|Texas Instruments Incorporated
|IWR6843AOP Single-Chip 60- to 64-GHz mmWave Sensor
[IBIS Ver]   4.1
[File name]   xwr6843aop_fcbga180.ibs
[Date]   04/01/2020
[File Rev]   1.0
[Source]
| Texas Instruments Incorporated.
| Analog-eLab Design Center, HPA
| 12500 TI Blvd
| Dallas, TX -75243
[Notes]   Revision History:
| Rev 1.0: 04/01/2020
| - Initial version of the model
| - C_comp although listed in numerical order of value are
|   obtained from varying PVT conditions. For PVT conditions for
|   each specific value refer the buffer description under
|   respective [Model]. IBIS model user is responsible for using
|   appropriate C_comp to simulate for Signal Integrity.
[Disclaimer]
| This model is designed as an aid for customers of Texas Instruments.
| TI and its licensors and suppliers make no warranties, either expressed
| or implied, with respect to this  model, including the warranties of
| merchantability or fitness for a particular purpose. The model is
| provided solely on an "as is" basis. The entire risk as to its quality
| and performance is with the customer.
| This model is subject to change without notice. Texas Instruments
| Incorporated is not responsible for updating this model.
[Copyright]
(C) Copyright 2018 Texas Instruments Incorporated.All rights reserved.
|  Component XI6843ARQGALP 180-pin FCBGA -ALP0180 package
|  Part # XI6843ARQGALP
[Component]   XI6843ARQGALP
[Manufacturer]   Texas Instruments
[Package]   |180 FCBGA - ALP0180 package
|  variable   typ   min   max
R_pkg   0.26   0.10   0.58
L_pkg   2.4nH   1.1nH   4.4nH
C_pkg   0.5pF   0.18pF   1.7pF
[Pin]   signal_name   model_name   R_pin   L_pin   C_pin
A1   VSS   GND   NA   NA   NA
A2   VSS   GND   NA   NA   NA
A3   DP11   IO1   NA   NA   NA
A4   DP13   IO1   NA   NA   NA
A5   VIN_SRAM   POWER   NA   NA   NA
A6   VSSA   GND   NA   NA   NA
A7   CLKP   NC   NA   NA   NA
A8   VSSA   GND   NA   NA   NA
A9   VOUT_14SYNTH   NC   NA   NA   NA
A10   VOUT_14APLL   NC   NA   NA   NA
A11   VSSA   GND   NA   NA   NA
A12   VIN_18VCO   POWER   NA   NA   NA
A13   VSSA   GND   NA   NA   NA
A14   OSC_CLKOUT   NC   NA   NA   NA
A15   VSSA   GND   NA   NA   NA
A16   VBGAP   NC   NA   NA   NA
A17   VSSA   GND   NA   NA   NA
A18   VSSA   GND   NA   NA   NA
B1   VIOIN_18   POWER   NA   NA   NA
B2   SPI_HOST_INTR   NC   NA   NA   NA
B3   DP9   IO1   NA   NA   NA
B4   DP12   IO1   NA   NA   NA
B5   DP15   IO1   NA   NA   NA
B6   VSSA   GND   NA   NA   NA
B7   CLKM   NC   NA   NA   NA
B8   VSSA   GND   NA   NA   NA
B9   VSSA   GND   NA   NA   NA
B10   VSSA   GND   NA   NA   NA
B11   VSSA   GND   NA   NA   NA
B12   VSSA   GND   NA   NA   NA
B13   VSSA   GND   NA   NA   NA
B14   VSSA   GND   NA   NA   NA
B15   VSSA   GND   NA   NA   NA
B16   VSSA   GND   NA   NA   NA
B17   VSSA   GND   NA   NA   NA
B18   VSSA   GND   NA   NA   NA
C1   VNWA   POWER   NA   NA   NA
C2   SPIA_CS_N   IO1   NA   NA   NA
C3   DP8   IO1   NA   NA   NA
C4   DP10   IO1   NA   NA   NA
C5   DP14   IO1   NA   NA   NA
C6   VSSA   GND   NA   NA   NA
C7   VSSA   GND   NA   NA   NA
C8   VSSA   GND   NA   NA   NA
C9   GPADC_5   NC   NA   NA   NA
C10   GPADC_6   NC   NA   NA   NA
C11   VIN_18VCO   POWER   NA   NA   NA
C12   VSSA   GND   NA   NA   NA
C13   VSSA   GND   NA   NA   NA
C14   VSSA   GND   NA   NA   NA
C15   VIN_18CLK   POWER   NA   NA   NA
C16   VSSA   GND   NA   NA   NA
C17   VSSA   GND   NA   NA   NA
C18   VIN_18CLK   POWER   NA   NA   NA
D1   SPIA_MISO   IO2   NA   NA   NA
D2   SPIA_CLK   IO2   NA   NA   NA
D3   SPIB_CS_N   IO2   NA   NA   NA
D16   VSSA   GND   NA   NA   NA
D17   VSSA   GND   NA   NA   NA
D18   VSSA   GND   NA   NA   NA
E1   VDDIN   POWER   NA   NA   NA
E2   SPIB_CLK   IO2   NA   NA   NA
E3   VSS   GND   NA   NA   NA
E16   VSSA   GND   NA   NA   NA
E17   VSSA   GND   NA   NA   NA
E18   VSSA   GND   NA   NA   NA
F1   VIOIN_18   POWER   NA   NA   NA
F2   SPIA_MOSI   IO2   NA   NA   NA
F3   VSS   GND   NA   NA   NA
F16   VSSA   GND   NA   NA   NA
F17   VSSA   GND   NA   NA   NA
F18   VSSA   GND   NA   NA   NA
G1   SPIB_MOSI   IO2   NA   NA   NA
G2   QSPI[1]   IO2   NA   NA   NA
G3   SPIB_MISO   IO2   NA   NA   NA
G16   VOUT_PA   NC   NA   NA   NA
G17   VOUT_PA   NC   NA   NA   NA
G18   VOUT_PA   NC   NA   NA   NA
H1   VIOIN   POWER   NA   NA   NA
H2   QSPI_CLK   IO2   NA   NA   NA
H3   QSPI[0]   IO2   NA   NA   NA
H16   VIN_13RF2   POWER   NA   NA   NA
H17   VIN_13RF2   POWER   NA   NA   NA
H18   VIN_13RF2   POWER   NA   NA   NA
J1   VDDIN   POWER   NA   NA   NA
J2   QSPI_CS_N   IO1   NA   NA   NA
J3   QSPI[2]   IO2   NA   NA   NA
J16   VIN_13RF1   POWER   NA   NA   NA
J17   VIN_13RF1   POWER   NA   NA   NA
J18   VIN_13RF1   POWER   NA   NA   NA
K1   VIOIN_18   POWER   NA   NA   NA
K2   QSPI[3]   IO2   NA   NA   NA
K3   GPIO_2   IO2   NA   NA   NA
K16   VSSA   GND   NA   NA   NA
K17   VSSA   GND   NA   NA   NA
K18   VSSA   GND   NA   NA   NA
L1   DP7   IO2   NA   NA   NA
L2   DP6   IO2   NA   NA   NA
L3   GPIO_1   IO2   NA   NA   NA
L16   VSSA   GND   NA   NA   NA
L17   VSSA   GND   NA   NA   NA
L18   VSSA   GND   NA   NA   NA
M1   DP5   IO2   NA   NA   NA
M2   GPIO_0   IO2   NA   NA   NA
M3   SYNC_OUT   IO2   NA   NA   NA
M16   VIN_18BB   POWER   NA   NA   NA
M17   VIN_18BB   POWER   NA   NA   NA
M18   VIN_18BB   POWER   NA   NA   NA
N1   LVDS_TXM[0]   ODF   NA   NA   NA
N2   LVDS_TXP[0]   ODF   NA   NA   NA
N3   VSS   GND   NA   NA   NA
N16   VSSA   GND   NA   NA   NA
N17   VSSA   GND   NA   NA   NA
N18   VSSA   GND   NA   NA   NA
P1   LVDS_TXM[1]   ODF   NA   NA   NA
P2   LVDS_TXP[1]   ODF   NA   NA   NA
P3   VSS   GND   NA   NA   NA
P16   VSSA   GND   NA   NA   NA
P17   GPADC_2   NC   NA   NA   NA
P18   GPADC_1   NC   NA   NA   NA
R1   LVDS_CLKP   ODF   NA   NA   NA
R2   LVDS_CLKM   ODF   NA   NA   NA
R3   VSS   GND   NA   NA   NA
R16   VSSA   GND   NA   NA   NA
R17   VSSA   GND   NA   NA   NA
R18   GPADC_3   NC   NA   NA   NA
T1   LVDS_FRCLKP   ODF   NA   NA   NA
T2   LVDS_FRCLKM   ODF   NA   NA   NA
T3   TCK   IO2   NA   NA   NA
T4   VSS   GND   NA   NA   NA
T5   VSS   GND   NA   NA   NA
T6   VSS   GND   NA   NA   NA
T7   VSS   GND   NA   NA   NA
T8   VSS   GND   NA   NA   NA
T9   VSS   GND   NA   NA   NA
T10   VSS   GND   NA   NA   NA
T11   VSS   GND   NA   NA   NA
T12   VSS   GND   NA   NA   NA
T13   VSS   GND   NA   NA   NA
T14   VSS   GND   NA   NA   NA
T15   VSS   GND   NA   NA   NA
T16   VSS   GND   NA   NA   NA
T17   VSSA   GND   NA   NA   NA
T18   GPADC_4   NC   NA   NA   NA
U1   VSS   GND   NA   NA   NA
U2   VIOIN_18DIFF   POWER   NA   NA   NA
U3   DMM_CLK   IO1   NA   NA   NA
U4   DMM_SYNC   IO1   NA   NA   NA
U5   DP3   IO1   NA   NA   NA
U6   DP1   IO1   NA   NA   NA
U7   DP0   IO1   NA   NA   NA
U8   TMS   IO1   NA   NA   NA
U9   TDI   IO1   NA   NA   NA
U10   TDO   IO1   NA   NA   NA
U11   NRESET   NC   NA   NA   NA
U12   SYNC_IN   IO1   NA   NA   NA
U13   WARM_RESET   IOOD   NA   NA   NA
U14   NERROR_IN   IOOD   NA   NA   NA
U15   NERROR_OUT   IOOD   NA   NA   NA
U16   RS232_TX   IO1   NA   NA   NA
U17   VSSA   GND   NA   NA   NA
U18   VSSA   GND   NA   NA   NA
V1   VSS   GND   NA   NA   NA
V2   VPP   POWER   NA   NA   NA
V3   DP4   IO1   NA   NA   NA
V4   VDDIN   POWER   NA   NA   NA
V5   DP2   IO1   NA   NA   NA
V6   VIN_SRAM   POWER   NA   NA   NA
V7   VNWA   POWER   NA   NA   NA
V8   VDDIN   POWER   NA   NA   NA
V9   VIOIN   POWER   NA   NA   NA
V10   PMIC_CLKOUT   IO1   NA   NA   NA
V11   VIOIN_18   POWER   NA   NA   NA
V12   VIN_SRAM   POWER   NA   NA   NA
V13   MCU_CLKOUT   IO1   NA   NA   NA
V14   VNWA   POWER   NA   NA   NA
V15   VDDIN   POWER   NA   NA   NA
V16   RS232_RX   IO1   NA   NA   NA
V17   VSSA   GND   NA   NA   NA
V18   VSSA   GND   NA   NA   NA
[Diff Pin]  inv_pin  vdiff  tdelay_typ  tdelay_min  tdelay_max
   N1   N2   0.1   NA   NA   NA
   P1   P2   0.1   NA   NA   NA
   R2   R1   0.1   NA   NA   NA
   T2   T1   0.1   NA   NA   NA
| Model IOOD
[Model Selector] IOOD
|SC1 IS A SLEW RATE CONTROL PIN
|5% SUPPLY VARIATION MODES WITH 1.8V NOM SUPPLY
IOOD_V_PUPDOFF_5P_SC1_1P8  Cell operated at 1.8(nom)
|IOOD_V_PUPDOFF_5P_SC1_1P8; BUFFER WITH WEAK PULUP/PULLDOWN OFF AT 5% SUPPLY
|VARIATION WITH SC1=1 MEANING SLOW MODE OF OPERATION
IOOD_V_PD_ON_5P_!SC1_1P8  Cell operated at 1.8(nom)
|IOOD_V_PD_ON_5P_!SC1_1P8; BUFFER WITH WEAK_PULLDOWN_ON AT 5% SUPPLY
|VARIATION WITH SC1=0 MEANING FAST MODE OF OPERATION
IOOD_V_PD_ON_5P_SC1_1P8  Cell operated at 1.8(nom)
|IOOD_V_PD_ON_5P_SC1_1P8; BUFFER WITH WEAK_PULLDOWN_ON AT 5% SUPPLY
|VARIATION WITH SC1=1 MEANING SLOW MODE OF OPERATION
IOOD_V_PU_ON_5P_!SC1_1P8  Cell operated at 1.8(nom)
|IOOD_V_PU_ON_5P_!SC1_1P8; BUFFER WITH WEAK_PULLUP_ON AT 5% SUPPLY
|VARIATION WITH SC1=0 MEANING FAST MODE OF OPERATION
IOOD_V_PUPDOFF_5P_!SC1_1P8  Cell operated at 1.8(nom)
|IOOD_V_PUPDOFF_5P_!SC1_1P8; BUFFER WITH WEAK PULUP/PULLDOWN OFF AT 5% SUPPLY
|VARIATION WITH SC1=0 MEANING FAST MODE OF OPERATION
IOOD_V_PU_ON_5P_SC1_1P8  Cell operated at 1.8(nom)
|IOOD_V_PU_ON_5P_SC1_1P8; BUFFER WITH WEAK_PULLUP_ON AT 5% SUPPLY
|VARIATION WITH SC1=1 MEANING SLOW MODE OF OPERATION
|5% SUPPLY VARIATION MODES WITH 3.3V NOM SUPPLY
IOOD_V_PUPDOFF_5P_SC1_3P3  Cell operated at 3.3(nom)
|IOOD_V_PUPDOFF_5P_SC1_3P3; BUFFER WITH WEAK PULUP/PULLDOWN OFF AT 5% SUPPLY
|VARIATION WITH SC1=1 MEANING SLOW MODE OF OPERATION
IOOD_V_PD_ON_5P_!SC1_3P3  Cell operated at 3.3(nom)
|IOOD_V_PD_ON_5P_!SC1_3P3; BUFFER WITH WEAK_PULLDOWN_ON AT 5% SUPPLY
|VARIATION WITH SC1=0 MEANING FAST MODE OF OPERATION
IOOD_V_PD_ON_5P_SC1_3P3  Cell operated at 3.3(nom)
|IOOD_V_PD_ON_5P_SC1_3P3; BUFFER WITH WEAK_PULLDOWN_ON AT 5% SUPPLY
|VARIATION WITH SC1=1 MEANING SLOW MODE OF OPERATION
IOOD_V_PU_ON_5P_!SC1_3P3  Cell operated at 3.3(nom)
|IOOD_V_PU_ON_5P_!SC1_3P3; BUFFER WITH WEAK_PULLUP_ON AT 5% SUPPLY
|VARIATION WITH SC1=0 MEANING FAST MODE OF OPERATION
IOOD_V_PUPDOFF_5P_!SC1_3P3  Cell operated at 3.3(nom)
|IOOD_V_PUPDOFF_5P_!SC1_3P3; BUFFER WITH WEAK PULUP/PULLDOWN OFF AT 5% SUPPLY
|VARIATION WITH SC1=0 MEANING FAST MODE OF OPERATION
IOOD_V_PU_ON_5P_SC1_3P3  Cell operated at 3.3(nom)
|IOOD_V_PU_ON_5P_SC1_3P3; BUFFER WITH WEAK_PULLUP_ON AT 5% SUPPLY
|VARIATION WITH SC1=1 MEANING SLOW MODE OF OPERATION
| 10% SUPPLY VARIATION MODES WITH 1.8V NOM SUPPLY
IOOD_V_PUPDOFF_10P_SC1_1P8  Cell operated at 1.8(nom)
|IOOD_V_PUPDOFF_10P_SC1_1P8; BUFFER WITH WEAK PULUP/PULLDOWN OFF AT 10% SUPPLY
|VARIATION WITH SC1=1 MEANING SLOW MODE OF OPERATION
IOOD_V_PD_ON_10P_!SC1_1P8  Cell operated at 1.8(nom)
|IOOD_V_PD_ON_10P_!SC1_1P8; BUFFER WITH WEAK_PULLDOWN_ON AT 10% SUPPLY
|VARIATION WITH SC1=0 MEANING FAST MODE OF OPERATION
IOOD_V_PD_ON_10P_SC1_1P8  Cell operated at 1.8(nom)
|IOOD_V_PD_ON_10P_SC1_1P8; BUFFER WITH WEAK_PULLDOWN_ON AT 10% SUPPLY
|VARIATION WITH SC1=1 MEANING SLOW MODE OF OPERATION
IOOD_V_PU_ON_10P_!SC1_1P8  Cell operated at 1.8(nom)
|IOOD_V_PU_ON_10P_!SC1_1P8; BUFFER WITH WEAK_PULLUP_ON AT 10% SUPPLY
|VARIATION WITH SC1=0 MEANING FAST MODE OF OPERATION
IOOD_V_PUPDOFF_10P_!SC1_1P8  Cell operated at 1.8(nom)
|IOOD_V_PUPDOFF_10P_!SC1_1P8; BUFFER WITH WEAK PULUP/PULLDOWN OFF AT 10% SUPPLY
|VARIATION WITH SC1=0 MEANING FAST MODE OF OPERATION
IOOD_V_PU_ON_10P_SC1_1P8  Cell operated at 1.8(nom)
|IOOD_V_PU_ON_10P_SC1_1P8; BUFFER WITH WEAK_PULLUP_ON AT 10% SUPPLY
|VARIATION WITH SC1=1 MEANING SLOW MODE OF OPERATION
| 10% SUPPLY VARIATION MODES WITH 3.3V NOM SUPPLY
IOOD_V_PUPDOFF_10P_SC1_3P3  Cell operated at 3.3(nom)
|IOOD_V_PUPDOFF_10P_SC1_3P3; BUFFER WITH WEAK PULUP/PULLDOWN OFF AT 10% SUPPLY
|VARIATION WITH SC1=1 MEANING SLOW MODE OF OPERATION
IOOD_V_PD_ON_10P_!SC1_3P3  Cell operated at 3.3(nom)
|IOOD_V_PD_ON_10P_!SC1_3P3; BUFFER WITH WEAK_PULLDOWN_ON 10% SUPPLY
|VARIATION WITH SC1=0 MEANING FAST MODE OF OPERATION
IOOD_V_PD_ON_10P_SC1_3P3  Cell operated at 3.3(nom)
|IOOD_V_PD_ON_10P_SC1_3P3; BUFFER WITH WEAK_PULLDOWN_ON AT 10% SUPPLY
|VARIATION WITH SC1=1 MEANING SLOW MODE OF OPERATION
IOOD_V_PU_ON_10P_!SC1_3P3  Cell operated at 3.3(nom)
|IOOD_V_PU_ON_10P_!SC1_3P3; BUFFER WITH WEAK_PULLUP_ON AT 10% SUPPLY
|VARIATION WITH SC1=0 MEANING FAST MODE OF OPERATION
IOOD_V_PUPDOFF_10P_!SC1_3P3  Cell operated at 3.3(nom)
|IOOD_V_PUPDOFF_10P_!SC1_3P3; BUFFER WITH WEAK PULUP/PULLDOWN OFF AT 10% SUPPLY
|VARIATION WITH SC1=0 MEANING FAST MODE OF OPERATION
IOOD_V_PU_ON_10P_SC1_3P3  Cell operated at 3.3(nom)
|IOOD_V_PU_ON_10P_SC1_3P3; BUFFER WITH WEAK_PULLUP_ON AT 10% SUPPLY
|VARIATION WITH SC1=1 MEANING SLOW MODE OF OPERATION
| Model IO1
[Model Selector] IO1
|SC1 IS A SLEW RATE CONTROL PIN
|5% SUPPLY VARIATION MODES WITH 1.8V NOM SUPPLY
IO1_V_PUPDOFF_5P_SC1_1P8  Cell operated at 1.8(nom)
|IO1_V_PUPDOFF_5P_SC1_1P8; BUFFER WITH WEAK PULUP/PULLDOWN OFF AT 5% SUPPLY
|VARIATION WITH SC1=1 MEANING SLOW MODE OF OPERATION
IO1_V_PD_ON_5P_!SC1_1P8  Cell operated at 1.8(nom)
|IO1_V_PD_ON_5P_!SC1_1P8; BUFFER WITH WEAK_PULLDOWN_ON AT 5% SUPPLY
|VARIATION WITH SC1=0 MEANING FAST MODE OF OPERATION
IO1_V_PD_ON_5P_SC1_1P8  Cell operated at 1.8(nom)
|IO1_V_PD_ON_5P_SC1_1P8; BUFFER WITH WEAK_PULLDOWN_ON AT 5% SUPPLY
|VARIATION WITH SC1=1 MEANING SLOW MODE OF OPERATION
IO1_V_PU_ON_5P_!SC1_1P8  Cell operated at 1.8(nom)
|IO1_V_PU_ON_5P_!SC1_1P8; BUFFER WITH WEAK_PULLUP_ON AT 5% SUPPLY
|VARIATION WITH SC1=0 MEANING FAST MODE OF OPERATION
IO1_V_PUPDOFF_5P_!SC1_1P8  Cell operated at 1.8(nom)
|IO1_V_PUPDOFF_5P_!SC1_1P8; BUFFER WITH WEAK PULUP/PULLDOWN OFF AT 5% SUPPLY
|VARIATION WITH SC1=0 MEANING FAST MODE OF OPERATION
IO1_V_PU_ON_5P_SC1_1P8  Cell operated at 1.8(nom)
|IO1_V_PU_ON_5P_SC1_1P8; BUFFER WITH WEAK_PULLUP_ON AT 5% SUPPLY
|VARIATION WITH SC1=1 MEANING SLOW MODE OF OPERATION
|5% SUPPLY VARIATION MODES WITH 3.3V NOM SUPPLY
IO1_V_PUPDOFF_5P_SC1_3P3  Cell operated at 3.3(nom)
|IO1_V_PUPDOFF_5P_SC1_3P3; BUFFER WITH WEAK PULUP/PULLDOWN OFF AT 5% SUPPLY
|VARIATION WITH SC1=1 MEANING SLOW MODE OF OPERATION
IO1_V_PD_ON_5P_!SC1_3P3  Cell operated at 3.3(nom)
|IO1_V_PD_ON_5P_!SC1_3P3; BUFFER WITH WEAK_PULLDOWN_ON AT 5% SUPPLY
|VARIATION WITH SC1=0 MEANING FAST MODE OF OPERATION
IO1_V_PD_ON_5P_SC1_3P3  Cell operated at 3.3(nom)
|IO1_V_PD_ON_5P_SC1_3P3; BUFFER WITH WEAK_PULLDOWN_ON AT 5% SUPPLY
|VARIATION WITH SC1=1 MEANING SLOW MODE OF OPERATION
IO1_V_PU_ON_5P_!SC1_3P3  Cell operated at 3.3(nom)
|IO1_V_PU_ON_5P_!SC1_3P3; BUFFER WITH WEAK_PULLUP_ON AT 5% SUPPLY
|VARIATION WITH SC1=0 MEANING FAST MODE OF OPERATION
IO1_V_PUPDOFF_5P_!SC1_3P3  Cell operated at 3.3(nom)
|IO1_V_PUPDOFF_5P_!SC1_3P3; BUFFER WITH WEAK PULUP/PULLDOWN OFF AT 5% SUPPLY
|VARIATION WITH SC1=0 MEANING FAST MODE OF OPERATION
IO1_V_PU_ON_5P_SC1_3P3  Cell operated at 3.3(nom)
|IO1_V_PU_ON_5P_SC1_3P3; BUFFER WITH WEAK_PULLUP_ON AT 5% SUPPLY
|VARIATION WITH SC1=1 MEANING SLOW MODE OF OPERATION
| 10% SUPPLY VARIATION MODES WITH 1.8V NOM SUPPLY
IO1_V_PUPDOFF_10P_SC1_1P8  Cell operated at 1.8(nom)
|IO1_V_PUPDOFF_10P_SC1_1P8; BUFFER WITH WEAK PULUP/PULLDOWN OFF AT 10% SUPPLY
|VARIATION WITH SC1=1 MEANING SLOW MODE OF OPERATION
IO1_V_PD_ON_10P_!SC1_1P8  Cell operated at 1.8(nom)
|IO1_V_PD_ON_10P_!SC1_1P8; BUFFER WITH WEAK_PULLDOWN_ON AT 10% SUPPLY
|VARIATION WITH SC1=0 MEANING FAST MODE OF OPERATION
IO1_V_PD_ON_10P_SC1_1P8  Cell operated at 1.8(nom)
|IO1_V_PD_ON_10P_SC1_1P8; BUFFER WITH WEAK_PULLDOWN_ON AT 10% SUPPLY
|VARIATION WITH SC1=1 MEANING SLOW MODE OF OPERATION
IO1_V_PU_ON_10P_!SC1_1P8  Cell operated at 1.8(nom)
|IO1_V_PU_ON_10P_!SC1_1P8; BUFFER WITH WEAK_PULLUP_ON AT 10% SUPPLY
|VARIATION WITH SC1=0 MEANING FAST MODE OF OPERATION
IO1_V_PUPDOFF_10P_!SC1_1P8  Cell operated at 1.8(nom)
|IO1_V_PUPDOFF_10P_!SC1_1P8; BUFFER WITH WEAK PULUP/PULLDOWN OFF AT 10% SUPPLY
|VARIATION WITH SC1=0 MEANING FAST MODE OF OPERATION
IO1_V_PU_ON_10P_SC1_1P8  Cell operated at 1.8(nom)
|IO1_V_PU_ON_10P_SC1_1P8; BUFFER WITH WEAK_PULLUP_ON AT 10% SUPPLY
|VARIATION WITH SC1=1 MEANING SLOW MODE OF OPERATION
| 10% SUPPLY VARIATION MODES WITH 3.3V NOM SUPPLY
IO1_V_PUPDOFF_10P_SC1_3P3  Cell operated at 3.3(nom)
|IO1_V_PUPDOFF_10P_SC1_3P3; BUFFER WITH WEAK PULUP/PULLDOWN OFF AT 10% SUPPLY
|VARIATION WITH SC1=1 MEANING SLOW MODE OF OPERATION
IO1_V_PD_ON_10P_!SC1_3P3  Cell operated at 3.3(nom)
|IO1_V_PD_ON_10P_!SC1_3P3; BUFFER WITH WEAK_PULLDOWN_ON 10% SUPPLY
|VARIATION WITH SC1=0 MEANING FAST MODE OF OPERATION
IO1_V_PD_ON_10P_SC1_3P3  Cell operated at 3.3(nom)
|IO1_V_PD_ON_10P_SC1_3P3; BUFFER WITH WEAK_PULLDOWN_ON AT 10% SUPPLY
|VARIATION WITH SC1=1 MEANING SLOW MODE OF OPERATION
IO1_V_PU_ON_10P_!SC1_3P3  Cell operated at 3.3(nom)
|IO1_V_PU_ON_10P_!SC1_3P3; BUFFER WITH WEAK_PULLUP_ON AT 10% SUPPLY
|VARIATION WITH SC1=0 MEANING FAST MODE OF OPERATION
IO1_V_PUPDOFF_10P_!SC1_3P3  Cell operated at 3.3(nom)
|IO1_V_PUPDOFF_10P_!SC1_3P3; BUFFER WITH WEAK PULUP/PULLDOWN OFF AT 10% SUPPLY
|VARIATION WITH SC1=0 MEANING FAST MODE OF OPERATION
IO1_V_PU_ON_10P_SC1_3P3  Cell operated at 3.3(nom)
|IO1_V_PU_ON_10P_SC1_3P3; BUFFER WITH WEAK_PULLUP_ON AT 10% SUPPLY
|VARIATION WITH SC1=1 MEANING SLOW MODE OF OPERATION
| Model IO2
[Model Selector] IO2
|SC1 IS A SLEW RATE CONTROL PIN
|5% SUPPLY VARIATION MODES WITH 1.8V NOM SUPPLY
IO2_H_PUPDOFF_5P_SC1_1P8  Cell operated at 1.8(nom)
|IO2_H_PUPDOFF_5P_SC1_1P8; BUFFER WITH WEAK PULUP/PULLDOWN OFF AT 5% SUPPLY
|VARIATION WITH SC1=1 MEANING SLOW MODE OF OPERATION
IO2_H_PD_ON_5P_!SC1_1P8  Cell operated at 1.8(nom)
|IO2_H_PD_ON_5P_!SC1_1P8; BUFFER WITH WEAK_PULLDOWN_ON AT 5% SUPPLY
|VARIATION WITH SC1=0 MEANING FAST MODE OF OPERATION
IO2_H_PD_ON_5P_SC1_1P8  Cell operated at 1.8(nom)
|IO2_H_PD_ON_5P_SC1_1P8; BUFFER WITH WEAK_PULLDOWN_ON AT 5% SUPPLY
|VARIATION WITH SC1=1 MEANING SLOW MODE OF OPERATION
IO2_H_PU_ON_5P_!SC1_1P8  Cell operated at 1.8(nom)
|IO2_H_PU_ON_5P_!SC1_1P8; BUFFER WITH WEAK_PULLUP_ON AT 5% SUPPLY
|VARIATION WITH SC1=0 MEANING FAST MODE OF OPERATION
IO2_H_PUPDOFF_5P_!SC1_1P8  Cell operated at 1.8(nom)
|IO2_H_PUPDOFF_5P_!SC1_1P8; BUFFER WITH WEAK PULUP/PULLDOWN OFF AT 5% SUPPLY
|VARIATION WITH SC1=0 MEANING FAST MODE OF OPERATION
IO2_H_PU_ON_5P_SC1_1P8  Cell operated at 1.8(nom)
|IO2_H_PU_ON_5P_SC1_1P8; BUFFER WITH WEAK_PULLUP_ON AT 5% SUPPLY
|VARIATION WITH SC1=1 MEANING SLOW MODE OF OPERATION
|5% SUPPLY VARIATION MODES WITH 3.3V NOM SUPPLY
IO2_H_PUPDOFF_5P_SC1_3P3  Cell operated at 3.3(nom)
|IO2_H_PUPDOFF_5P_SC1_3P3; BUFFER WITH WEAK PULUP/PULLDOWN OFF AT 5% SUPPLY
|VARIATION WITH SC1=1 MEANING SLOW MODE OF OPERATION
IO2_H_PD_ON_5P_!SC1_3P3  Cell operated at 3.3(nom)
|IO2_H_PD_ON_5P_!SC1_3P3; BUFFER WITH WEAK_PULLDOWN_ON AT 5% SUPPLY
|VARIATION WITH SC1=0 MEANING FAST MODE OF OPERATION
IO2_H_PD_ON_5P_SC1_3P3  Cell operated at 3.3(nom)
|IO2_H_PD_ON_5P_SC1_3P3; BUFFER WITH WEAK_PULLDOWN_ON AT 5% SUPPLY
|VARIATION WITH SC1=1 MEANING SLOW MODE OF OPERATION
IO2_H_PU_ON_5P_!SC1_3P3  Cell operated at 3.3(nom)
|IO2_H_PU_ON_5P_!SC1_3P3; BUFFER WITH WEAK_PULLUP_ON AT 5% SUPPLY
|VARIATION WITH SC1=0 MEANING FAST MODE OF OPERATION
IO2_H_PUPDOFF_5P_!SC1_3P3  Cell operated at 3.3(nom)
|IO2_H_PUPDOFF_5P_!SC1_3P3; BUFFER WITH WEAK PULUP/PULLDOWN OFF AT 5% SUPPLY
|VARIATION WITH SC1=0 MEANING FAST MODE OF OPERATION
IO2_H_PU_ON_5P_SC1_3P3  Cell operated at 3.3(nom)
|IO2_H_PU_ON_5P_SC1_3P3; BUFFER WITH WEAK_PULLUP_ON AT 5% SUPPLY
|VARIATION WITH SC1=1 MEANING SLOW MODE OF OPERATION
| 10% SUPPLY VARIATION MODES WITH 1.8V NOM SUPPLY
IO2_H_PUPDOFF_10P_SC1_1P8  Cell operated at 1.8(nom)
|IO2_H_PUPDOFF_10P_SC1_1P8; BUFFER WITH WEAK PULUP/PULLDOWN OFF AT 10% SUPPLY
|VARIATION WITH SC1=1 MEANING SLOW MODE OF OPERATION
IO2_H_PD_ON_10P_!SC1_1P8  Cell operated at 1.8(nom)
|IO2_H_PD_ON_10P_!SC1_1P8; BUFFER WITH WEAK_PULLDOWN_ON AT 10% SUPPLY
|VARIATION WITH SC1=0 MEANING FAST MODE OF OPERATION
IO2_H_PD_ON_10P_SC1_1P8  Cell operated at 1.8(nom)
|IO2_H_PD_ON_10P_SC1_1P8; BUFFER WITH WEAK_PULLDOWN_ON AT 10% SUPPLY
|VARIATION WITH SC1=1 MEANING SLOW MODE OF OPERATION
IO2_H_PU_ON_10P_!SC1_1P8  Cell operated at 1.8(nom)
|IO2_H_PU_ON_10P_!SC1_1P8; BUFFER WITH WEAK_PULLUP_ON AT 10% SUPPLY
|VARIATION WITH SC1=0 MEANING FAST MODE OF OPERATION
IO2_H_PUPDOFF_10P_!SC1_1P8  Cell operated at 1.8(nom)
|IO2_H_PUPDOFF_10P_!SC1_1P8; BUFFER WITH WEAK PULUP/PULLDOWN OFF AT 10% SUPPLY
|VARIATION WITH SC1=0 MEANING FAST MODE OF OPERATION
IO2_H_PU_ON_10P_SC1_1P8  Cell operated at 1.8(nom)
|IO2_H_PU_ON_10P_SC1_1P8; BUFFER WITH WEAK_PULLUP_ON AT 10% SUPPLY
|VARIATION WITH SC1=1 MEANING SLOW MODE OF OPERATION
| 10% SUPPLY VARIATION MODES WITH 3.3V NOM SUPPLY
IO2_H_PUPDOFF_10P_SC1_3P3  Cell operated at 3.3(nom)
|IO2_H_PUPDOFF_10P_SC1_3P3; BUFFER WITH WEAK PULUP/PULLDOWN OFF AT 10% SUPPLY
|VARIATION WITH SC1=1 MEANING SLOW MODE OF OPERATION
IO2_H_PD_ON_10P_!SC1_3P3  Cell operated at 3.3(nom)
|IO2_H_PD_ON_10P_!SC1_3P3; BUFFER WITH WEAK_PULLDOWN_ON 10% SUPPLY
|VARIATION WITH SC1=0 MEANING FAST MODE OF OPERATION
IO2_H_PD_ON_10P_SC1_3P3  Cell operated at 3.3(nom)
|IO2_H_PD_ON_10P_SC1_3P3; BUFFER WITH WEAK_PULLDOWN_ON AT 10% SUPPLY
|VARIATION WITH SC1=1 MEANING SLOW MODE OF OPERATION
IO2_H_PU_ON_10P_!SC1_3P3  Cell operated at 3.3(nom)
|IO2_H_PU_ON_10P_!SC1_3P3; BUFFER WITH WEAK_PULLUP_ON AT 10% SUPPLY
|VARIATION WITH SC1=0 MEANING FAST MODE OF OPERATION
IO2_H_PUPDOFF_10P_!SC1_3P3  Cell operated at 3.3(nom)
|IO2_H_PUPDOFF_10P_!SC1_3P3; BUFFER WITH WEAK PULUP/PULLDOWN OFF AT 10% SUPPLY
|VARIATION WITH SC1=0 MEANING FAST MODE OF OPERATION
IO2_H_PU_ON_10P_SC1_3P3  Cell operated at 3.3(nom)
|IO2_H_PU_ON_10P_SC1_3P3; BUFFER WITH WEAK_PULLUP_ON AT 10% SUPPLY
|VARIATION WITH SC1=1 MEANING SLOW MODE OF OPERATION
| Model ODF
[Model Selector] ODF
ODF_MODE_10P_1P8  Cell operated at 1.8(nom)
|ODF_MODE_10P_1P8; LVDS DRIVER MODE WITH 10PER VDDS
ODF_MODE_5P_1P8  Cell operated at 1.8(nom)
[Define Package Model]   XI6843ARQGALP
[Manufacturer]   TI
[OEM]   TI
[Description]   FCBGA
|[Number of Sections]   1
[Number of Pins]   67
[Pin Numbers]
|[Pin Name]  Net Number   Net Name   Net's All Pins
B7   | 1   CLKM   B7
A7   | 2   CLKP   A7
U3   | 3   DMM_CLK   U3
U4   | 4   DMM_SYNC   U4
U7   | 5   DP0   U7
U6   | 6   DP1   U6
V5   | 7   DP2   V5
U5   | 8   DP3   U5
V3   | 9   DP4   V3
M1   | 10   DP5   M1
L2   | 11   DP6   L2
L1   | 12   DP7   L1
C3   | 13   DP8   C3
B3   | 14   DP9   B3
C4   | 15   DP10   C4
A3   | 16   DP11   A3
B4   | 17   DP12   B4
A4   | 18   DP13   A4
C5   | 19   DP14   C5
B5   | 20   DP15   B5
P18   | 21   GPADC_1   P18
P17   | 22   GPADC_2   P17
R18   | 23   GPADC_3   R18
T18   | 24   GPADC_4   T18
C9   | 25   GPADC_5   C9
C10   | 26   GPADC_6   C10
M2   | 27   GPIO_0   M2
L3   | 28   GPIO_1   L3
K3   | 29   GPIO_2   K3
R2   | 30   LVDS_CLKM   R2
R1   | 31   LVDS_CLKP   R1
T2   | 32   LVDS_FRCLKM   T2
T1   | 33   LVDS_FRCLKP   T1
N1   | 34   LVDS_TXM_0   N1
P1   | 35   LVDS_TXM_1   P1
N2   | 36   LVDS_TXP_0   N2
P2   | 37   LVDS_TXP_1   P2
V13   | 38   MCU_CLKOUT   V13
D1   | 39   MISO_1   D1
G3   | 40   MISO_2   G3
F2   | 41   MOSI_1   F2
G1   | 42   MOSI_2   G1
U14   | 43   NERROR_IN   U14
U15   | 44   NERROR_OUT   U15
U11   | 45   NRESET   U11
A14   | 46   OSC_CLKOUT   A14
V10   | 47   PMIC_CLKOUT   V10
H3   | 48   QSPI_0   H3
G2   | 49   QSPI_1   G2
J3   | 50   QSPI_2   J3
K2   | 51   QSPI_3   K2
H2   | 52   QSPI_CLK   H2
J2   | 53   QSPI_CS   J2
V16   | 54   RS232_RX   V16
U16   | 55   RS232_TX   U16
D2   | 56   SPI_CLK_1   D2
E2   | 57   SPI_CLK_2   E2
C2   | 58   SPI_CS_1   C2
D3   | 59   SPI_CS_2   D3
B2   | 60   SPI_HOST_INTR_1   B2
U12   | 61   SYNC_IN   U12
M3   | 62   SYNC_OUT   M3
T3   | 63   TCK   T3
U9   | 64   TDI   U9
U10   | 65   TDO   U10
U8   | 66   TMS   U8
U13   | 67   WARM_RESET   U13
[Model Data]
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[End Model Data]
[End Package Model]
| Models and submodels in the file (74): IOOD_V_PUPDOFF_5P_SC1_1P8 (I/O_open_drain), IOOD_V_PD_ON_5P_!SC1_1P8 (I/O_open_drain), IOOD_V_PD_ON_5P_SC1_1P8 (I/O_open_drain), IOOD_V_PU_ON_5P_!SC1_1P8 (I/O_open_drain), IOOD_V_PUPDOFF_5P_!SC1_1P8 (I/O_open_drain), IOOD_V_PU_ON_5P_SC1_1P8 (I/O_open_drain), IOOD_V_PUPDOFF_5P_SC1_3P3 (I/O_open_drain), IOOD_V_PD_ON_5P_!SC1_3P3 (I/O_open_drain), IOOD_V_PD_ON_5P_SC1_3P3 (I/O_open_drain), IOOD_V_PU_ON_5P_!SC1_3P3 (I/O_open_drain), IOOD_V_PUPDOFF_5P_!SC1_3P3 (I/O_open_drain), IOOD_V_PU_ON_5P_SC1_3P3 (I/O_open_drain), IOOD_V_PUPDOFF_10P_SC1_1P8 (I/O_open_drain), IOOD_V_PD_ON_10P_!SC1_1P8 (I/O_open_drain), IOOD_V_PD_ON_10P_SC1_1P8 (I/O_open_drain), IOOD_V_PU_ON_10P_!SC1_1P8 (I/O_open_drain), IOOD_V_PUPDOFF_10P_!SC1_1P8 (I/O_open_drain), IOOD_V_PU_ON_10P_SC1_1P8 (I/O_open_drain), IOOD_V_PUPDOFF_10P_SC1_3P3 (I/O_open_drain), IOOD_V_PD_ON_10P_!SC1_3P3 (I/O_open_drain), IOOD_V_PD_ON_10P_SC1_3P3 (I/O_open_drain), IOOD_V_PU_ON_10P_!SC1_3P3 (I/O_open_drain), IOOD_V_PUPDOFF_10P_!SC1_3P3 (I/O_open_drain), IOOD_V_PU_ON_10P_SC1_3P3 (I/O_open_drain), IO1_V_PUPDOFF_5P_SC1_1P8 (I/O), IO1_V_PD_ON_5P_!SC1_1P8 (I/O), IO1_V_PD_ON_5P_SC1_1P8 (I/O), IO1_V_PU_ON_5P_!SC1_1P8 (I/O), IO1_V_PUPDOFF_5P_!SC1_1P8 (I/O), IO1_V_PU_ON_5P_SC1_1P8 (I/O), IO1_V_PUPDOFF_5P_SC1_3P3 (I/O), IO1_V_PD_ON_5P_!SC1_3P3 (I/O), IO1_V_PD_ON_5P_SC1_3P3 (I/O), IO1_V_PU_ON_5P_!SC1_3P3 (I/O), IO1_V_PUPDOFF_5P_!SC1_3P3 (I/O), IO1_V_PU_ON_5P_SC1_3P3 (I/O), IO1_V_PUPDOFF_10P_SC1_1P8 (I/O), IO1_V_PD_ON_10P_!SC1_1P8 (I/O), IO1_V_PD_ON_10P_SC1_1P8 (I/O), IO1_V_PU_ON_10P_!SC1_1P8 (I/O), IO1_V_PUPDOFF_10P_!SC1_1P8 (I/O), IO1_V_PU_ON_10P_SC1_1P8 (I/O), IO1_V_PUPDOFF_10P_SC1_3P3 (I/O), IO1_V_PD_ON_10P_!SC1_3P3 (I/O), IO1_V_PD_ON_10P_SC1_3P3 (I/O), IO1_V_PU_ON_10P_!SC1_3P3 (I/O), IO1_V_PUPDOFF_10P_!SC1_3P3 (I/O), IO1_V_PU_ON_10P_SC1_3P3 (I/O), IO2_H_PUPDOFF_5P_SC1_1P8 (I/O), IO2_H_PD_ON_5P_!SC1_1P8 (I/O), IO2_H_PD_ON_5P_SC1_1P8 (I/O), IO2_H_PU_ON_5P_!SC1_1P8 (I/O), IO2_H_PUPDOFF_5P_!SC1_1P8 (I/O), IO2_H_PU_ON_5P_SC1_1P8 (I/O), IO2_H_PUPDOFF_5P_SC1_3P3 (I/O), IO2_H_PD_ON_5P_!SC1_3P3 (I/O), IO2_H_PD_ON_5P_SC1_3P3 (I/O), IO2_H_PU_ON_5P_!SC1_3P3 (I/O), IO2_H_PUPDOFF_5P_!SC1_3P3 (I/O), IO2_H_PU_ON_5P_SC1_3P3 (I/O), IO2_H_PUPDOFF_10P_SC1_1P8 (I/O), IO2_H_PD_ON_10P_!SC1_1P8 (I/O), IO2_H_PD_ON_10P_SC1_1P8 (I/O), IO2_H_PU_ON_10P_!SC1_1P8 (I/O), IO2_H_PUPDOFF_10P_!SC1_1P8 (I/O), IO2_H_PU_ON_10P_SC1_1P8 (I/O), IO2_H_PUPDOFF_10P_SC1_3P3 (I/O), IO2_H_PD_ON_10P_!SC1_3P3 (I/O), IO2_H_PD_ON_10P_SC1_3P3 (I/O), IO2_H_PU_ON_10P_!SC1_3P3 (I/O), IO2_H_PUPDOFF_10P_!SC1_3P3 (I/O), IO2_H_PU_ON_10P_SC1_3P3 (I/O), ODF_MODE_10P_1P8 (3-state), ODF_MODE_5P_1P8 (3-state)
